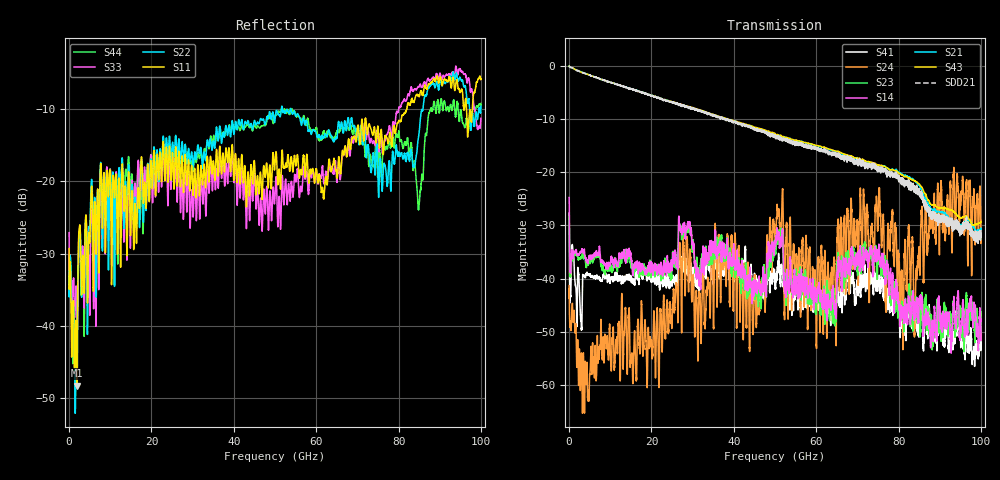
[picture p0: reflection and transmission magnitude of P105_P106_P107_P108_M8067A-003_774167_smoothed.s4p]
!Keysight Technologies PLTS 2021(64 bit), Build 20210202.1
!S11 smoothed in format LOGMAG, average points = 21
!S12 smoothed in format LOGMAG, average points = 21
!S13 smoothed in format LOGMAG, average points = 21
!S14 smoothed in format LOGMAG, average points = 21
!S21 smoothed in format LOGMAG, average points = 21
!S22 smoothed in format LOGMAG, average points = 21
!S23 smoothed in format LOGMAG, average points = 21
!S24 smoothed in format LOGMAG, average points = 21
!S31 smoothed in format LOGMAG, average points = 21
!S32 smoothed in format LOGMAG, average points = 21
!S33 smoothed in format LOGMAG, average points = 21
!S34 smoothed in format LOGMAG, average points = 21
!S41 smoothed in format LOGMAG, average points = 21
!S42 smoothed in format LOGMAG, average points = 21
!S43 smoothed in format LOGMAG, average points = 21
!S44 smoothed in format LOGMAG, average points = 21
!$DUT_CFG_DESC: Default 4-Port Configuration
!$NUMBER_PORTS: 4
!$DIFF_PORT_MAP: 1|2P|2|2P|0|UC|0|UC|
!$PORT_MAP: 1|1|<<<<<<|2|2|>>>>>>|3|3|<<<<<<|4|4|>>>>>>|
!Date: Monday, December 04, 2023, 05:54:12
!S4P File: Measurements: <S11,S12,S13,S14>,
!<S21,S22,S23,S24>,
!<S31,S32,S33,S34>,
!<S41,S42,S43,S44>:
# MHz S  RI  R 50
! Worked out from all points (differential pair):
!   10000 points, 10 MHz to 100 GHz, reference 50 ohm
!   strongest paths, dB at 10 MHz, 25.01 GHz, 50.01 GHz, 75.01 GHz, 100 GHz:
!     S43: -0.1, -6.8, -12.8, -18.6, -29.4
!     S21: -0.1, -6.8, -12.9, -18.7, -30.5
!     S14: -24.8, -37.8, -32.8, -36.3, -51.7
!     S23: -28.6, -36.7, -34.8, -36.8, -47.4
!     S24: -41.3, -48.4, -32.2, -30.4, -33.0
!     S41: -27.7, -41.1, -40.8, -40.6, -49.4
!   taken as a pair (ports 3,1 in; 4,2 out), SDD21 dB: -0.1, -6.9, -13.4, -19.2, -31.8
!   lowest |S11| = -48.2 dB at 1.84 GHz (marker M1), VSWR 1.01, Z = 50.1 - j0.371 ohm
!   |S11| at or under -10 dB: start of sweep to 82.03 GHz; 95.85344 GHz to 95.92746 GHz (74.02 MHz wide, 0.0772 % of centre); 96.52 GHz to 97.92 GHz (1.402 GHz wide, 1.44 % of centre)
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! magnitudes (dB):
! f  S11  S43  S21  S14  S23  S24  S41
! 10 MHz  -29.3  -0.1  -0.1  -24.8  -28.6  -41.3  -27.7
! 1.84 GHz  -48.2  -0.9  -0.8  -35.2  -35.8  -56.2  -46.4
! 23.23 GHz  -19.8  -6.3  -6.4  -38.6  -36.9  -49.7  -40.0
! 75.01 GHz  -12.5  -18.6  -18.7  -36.3  -36.8  -30.4  -40.6
! 80.78 GHz  -11.1  -20.6  -20.4  -47.2  -45.4  -38.8  -48.3
! 95.2 GHz  -7.4  -28.6  -30.0  -48.5  -46.9  -23.9  -50.1
! 100 GHz  -5.8  -29.4  -30.5  -51.7  -47.4  -33.0  -49.4
